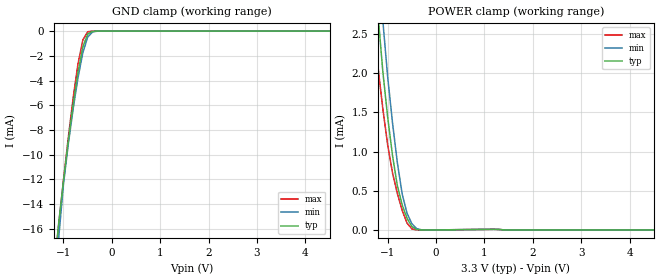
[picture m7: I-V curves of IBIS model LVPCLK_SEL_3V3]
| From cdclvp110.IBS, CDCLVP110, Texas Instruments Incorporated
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|   Clock Select Input  Model for 3.3V VCC range   |
[Model]   LVPCLK_SEL_3V3
Model_type   Input
| Signals   CLK_SEL
| variable   typ   min   max
C_comp   0.5pF   NA   NA
Vinl = 1.825V   | VCC-1.475 (max)
Vinh = 2.135V   | VCC-1.165 (min)
[Model Spec]
|   VCC=3.3V   VCC=3.0V   VCC=3.8V
Vinl   1.825V   1.525V   2.325V
Vinh   2.135V   1.835V   2.635V
[Temperature Range]   40C   110C   -40C
[Voltage range]   3.3V   3.0V   3.8V
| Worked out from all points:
|   GND clamp passes 1 mA (typ) near -0.57 V on its own axis
|   POWER clamp passes 1 mA (typ) near -0.91 V on its own axis
[POWER Clamp]
|   40C:3.3V:nominal   110C:3.0V:weak   -40C:3.8:strong
|  Voltage   I(typ)   I(min)   I(max)
-3.9V     152.3mA    160.9mA    153.3mA
-1.3V     3.667mA    4.676mA    2.791mA
-1.2V     2.745mA    3.584mA    2.076mA
-1.1V     2.017mA    2.664mA    1.543mA
-1V       1.437mA    1.95mA     1.084mA
-900mV    947.5uA    1.365mA    726.2uA
-800mV    563.8uA    857uA      464.8uA
-700mV    317.2uA    457.4uA    248.2uA
-600mV    149.5uA    212.6uA    88.33uA
-500mV    42.85uA    79.46uA    12.41uA
-200mV    9.389nA    123.9nA    630.5pA
7.6V      0A         0A         0A
[GND Clamp]
|   40C:3.3V:nominal   110C:3.0V:weak   -40C:3.8:strong
|  Voltage   I(typ)   I(min)   I(max)
-3.8V     -231.9mA   -260.1mA   -206.1mA
-1.2V     -19.64mA   -22.93mA   -19.53mA
-1.1V     -15.55mA   -16.76mA   -15.72mA
-1V       -12.09mA   -12.38mA   -12.06mA
-900mV    -8.882mA   -9.114mA   -8.599mA
-800mV    -5.924mA   -6.282mA   -5.407mA
-700mV    -3.314mA   -3.777mA   -2.651mA
-600mV    -1.29mA    -1.749mA   -715uA
-500mV    -238.7uA   -492.2uA   -55.21uA
-400mV    -19.24uA   -71.63uA   -1.479uA
-200mV    -34.19nA   -474nA     -355.3pA
7.6V      0A         0A         0A
